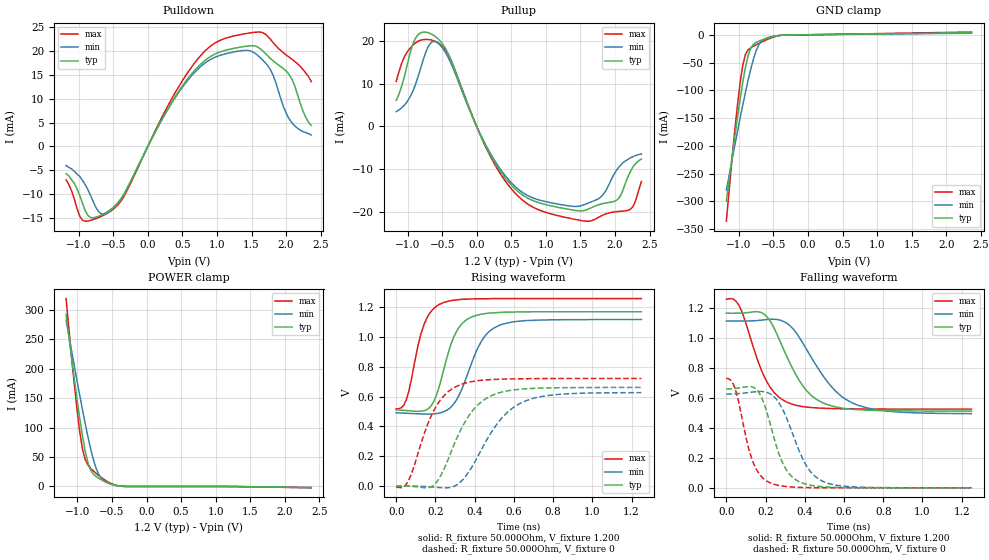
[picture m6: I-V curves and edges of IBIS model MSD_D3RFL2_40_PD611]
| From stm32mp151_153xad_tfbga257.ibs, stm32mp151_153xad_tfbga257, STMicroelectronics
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[Model] MSD_D3RFL2_40_PD611
Model_type   I/O
C_comp 2.448pF   2.362pF   2.573pF
Vinh = 820.000mV
Vinl = 380.000mV
Vmeas = 600.000mV
Vref = 600.000mV
[Model Spec]
Vinh   820.000mV   790.000mV   870.000mV
Vinl   380.000mV   350.000mV   430.000mV
Vmeas   600.000mV   570.000mV   650.000mV
Vref   600.000mV   570.000mV   650.000mV
[Temperature Range]   25.000   125.000   -40.000
[Voltage Range]   1.200V   1.140V   1.300V
[GND Clamp Reference]   0.00V   0.00V   0.00V
[Pulldown Reference]   0.00V   0.00V   0.00V
[POWER Clamp Reference]   1.200V   1.140V   1.300V
[Pullup Reference]   1.200V   1.140V   1.300V
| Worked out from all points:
|   slope of the pulldown table from 0 to 0.18 V, typ, clamps not added: 35.6 ohm
|   slope of the pullup table from 0 to 0.18 V, typ, clamps not added: 29.6 ohm
|   GND clamp passes 1 mA (typ) near -0.40 V on its own axis
|   POWER clamp passes 1 mA (typ) near -0.41 V on its own axis
|   rising waveform, R_fixture 50.000Ohm, V_fixture 1.200: 20-80 % time 94.5ps typ, 122ps min, 81.1ps max; typ from 0.51 V to 1.17 V
|   rising waveform, R_fixture 50.000Ohm, V_fixture 0: 20-80 % time 155ps typ, 188ps min, 132ps max; typ from 0.001 V to 0.661 V
|   falling waveform, R_fixture 50.000Ohm, V_fixture 1.200: 20-80 % time 159ps typ, 201ps min, 127ps max; typ from 1.17 V to 0.512 V
|   falling waveform, R_fixture 50.000Ohm, V_fixture 0: 20-80 % time 99.9ps typ, 124ps min, 84ps max; typ from 0.66 V to 0 V
[GND Clamp]
-1.182V   -299.5mA   -279.6mA   -335.7mA
-1.064V   -187.3mA   -201.7mA   -177.4mA
-984.9mV  -117.8mA   -151.5mA   -88.49mA
-945.5mV  -86.46mA   -127.3mA   -55.67mA
-906.1mV  -59.05mA   -103.8mA   -35.55mA
-866.7mV  -37.55mA   -81.66mA   -27.13mA
-827.3mV  -23.74mA   -61.1mA    -23.33mA
-748.5mV  -13.56mA   -28.1mA    -17.89mA
-709.1mV  -11.37mA   -17.48mA   -15.38mA
-630.3mV  -7.842mA   -7.517mA   -10.66mA
-472.7mV  -2.44mA    -2.145mA   -3.165mA
2.364V    3.741mA    2.874mA    4.907mA
[Power Clamp]
-1.164V   292.4mA    282.5mA    319.2mA
-1.085V   218.6mA    230.8mA    220mA
-1.006V   148.4mA    180mA      131.1mA
-966.7mV  115.9mA    155.1mA    93.3mA
-927.3mV  86.08mA    130.8mA    63.93mA
-887.9mV  60.35mA    107.3mA    45.81mA
-809.1mV  27.78mA    64.27mA    31.09mA
-730.3mV  17.01mA    31.11mA    22.38mA
-690.9mV  13.91mA    20.28mA    18.51mA
-572.7mV  6.625mA    6.535mA    8.753mA
-336.4mV  188.6uA    356.2uA    213.6uA
2.382V    -1.927mA   -1.589mA   -2.285mA
[Pulldown]
-1.182V   -5.7mA     -4mA       -7mA
-945.5mV  -11.89mA   -7.1mA     -15.47mA
-866.7mV  -14.47mA   -9.06mA    -15.66mA
-709.1mV  -14.63mA   -13.73mA   -14.89mA
-551.5mV  -13.37mA   -13.66mA   -13.72mA
-354.6mV  -10.22mA   -10.3mA    -10.71mA
590.9mV   14.46mA    14.13mA    15.79mA
945.5mV   19.18mA    18.53mA    21.45mA
1.339V    20.84mA    20.05mA    23.48mA
1.733V    19.02mA    16.98mA    23.14mA
2.009V    15.7mA     6.74mA     19.1mA
2.364V    4.4mA      2.4mA      13.6mA
[Pullup]
-1.164V   6.1mA      3.457mA    10.51mA
-887.9mV  20.5mA     9.662mA    19.46mA
-730.3mV  21.97mA    17.57mA    20.3mA
-612.1mV  21.14mA    19.85mA    19.93mA
-375.8mV  15.68mA    14.87mA    15.59mA
215.2mV   -7.105mA   -6.743mA   -7.481mA
687.9mV   -16.23mA   -15.64mA   -17.48mA
1.476V    -19.64mA   -18.59mA   -21.81mA
1.791V    -18.11mA   -16.51mA   -20.92mA
1.988V    -17.46mA   -11.08mA   -19.91mA
2.264V    -9.3mA     -6.995mA   -18.58mA
2.382V    -7.6mA     -6.395mA   -12.82mA
[Ramp]
R_load=50.000Ohm
dV/dt_r   394.770mV/125.500ps  374.219mV/156.000ps  434.940mV/106.500ps
dV/dt_f   394.770mV/130.000ps  374.219mV/164.500ps  434.940mV/105.500ps
[Rising waveform]
R_fixture=50.000Ohm
V_fixture=1.200
V_fixture_min=1.140
V_fixture_max=1.300
0s        510.4mV    490.8mV    517.4mV
52ps      506.2mV    487.9mV    579.2mV
141ps     504.6mV    482.7mV    1.079V
179ps     539.2mV    482.6mV    1.171V
218ps     660.8mV    488.6mV    1.215V
281ps     956.5mV    531.9mV    1.242V
332ps     1.082V     640.8mV    1.25V
435ps     1.151V     970.7mV    1.254V
524ps     1.162V     1.075V     1.255V
1.25ns    1.167V     1.115V     1.255V
[Rising waveform]
R_fixture=50.000Ohm
V_fixture=0
0s        809.4uV    799uV      -5.389mV
64ps      36.01uV    794.3uV    41.16mV
192ps     6.778mV    -6.334mV   506.5mV
243ps     112.5mV    -11.03mV   604mV
320ps     352.9mV    19.62mV    675.3mV
447ps     576.6mV    275.4mV    710mV
537ps     629mV      453.8mV    716mV
626ps     647.9mV    550.2mV    718.4mV
830ps     658.6mV    614.3mV    720.3mV
1.25ns    660.9mV    625.8mV    720.6mV
[Falling waveform]
R_fixture=50.000Ohm
V_fixture=1.200
V_fixture_min=1.140
V_fixture_max=1.300
0s        1.167V     1.114V     1.26V
64ps      1.167V     1.114V     1.22V
192ps     1.161V     1.122V     745.9mV
243ps     1.068V     1.126V     637mV
307ps     881.3mV    1.101V     573.6mV
435ps     614.9mV    867.3mV    536.2mV
537ps     547.2mV    674.6mV    529.8mV
639ps     524.9mV    569.8mV    527.3mV
843ps     514.8mV    510mV      526.1mV
1.25ns    512.2mV    495.3mV    526mV
[Falling waveform]
R_fixture=50.000Ohm
V_fixture=0
0s        660.4mV    625.9mV    731.1mV
52ps      664.7mV    628.5mV    632mV
141ps     670.1mV    640.9mV    156.3mV
179ps     606mV      643.6mV    74.67mV
218ps     454mV      631.8mV    36.79mV
269ps     224mV      566.7mV    15.6mV
320ps     94.78mV    424.5mV    6.885mV
409ps     23.22mV    146.1mV    1.677mV
498ps     6.9mV      40.09mV    451.5uV
1.25ns    3.354uV    26.25uV    1.109uV
